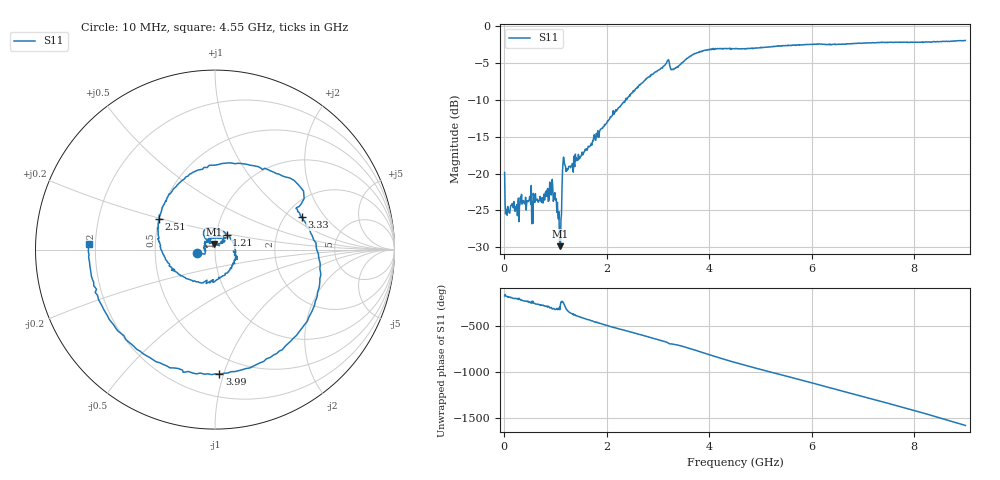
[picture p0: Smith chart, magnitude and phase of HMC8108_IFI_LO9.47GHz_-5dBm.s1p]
! Analog Devices, Inc.
! 1 Analog Way
! Wilmington, MA 01887
! http://www.analog.com
! Date:  2021-09-07 NN
! Board Name:  EV1HMC8108LC5 Revision A with HMC8108LC5 installed
! File Description:  S-Parameters for evaluation board without connectors or board loss de-embedded
! File Generation:  Calibrated Network Analyzer
! Chip Part Number:  HMC8108
! Chip Description:  X-Band, GaAs, MMIC, Low Noise Converter
! Chip Frequency:  9 to 10 GHz
! Chip Package:  LCC, 5 x 5 x 1.12 mm
! Chip State:
!  Temperature:  25C
!  LO Frequency:  9.47GHz
!  LO Power:  -5dBm
! Note:
!  Analog Devices supplies this data as a sample of measured data at the evaluation board
!  ports for this product.  Your particular data for this product may vary.
!  Analog Devices reserves the right to change this data at anytime.
!  All lines below in this file are as is from the Network Analyzer.
!Keysight Technologies,N5245A,MY49151104,A.10.65.16
!Date: Thursday, August 19, 2021 13:48:33
!Correction: S22(Full 2 Port(1,2))
!S1P File: Measurement: S22:
# Hz S  dB  R 50
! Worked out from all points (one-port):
!   900 points, 10 MHz to 9 GHz, reference 50 ohm
!   lowest |S11| = -29.8 dB at 1.1 GHz (marker M1), VSWR 1.07, Z = 49.4 + j3.15 ohm
!   |S11| at or under -10 dB: start of sweep to 2.373 GHz
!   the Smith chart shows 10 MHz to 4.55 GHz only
!   S11 on the Smith chart (normalised r, x): 10 MHz: 0.82, -0.03; 1.21 GHz: 1.12, +0.18; 2.51 GHz: 0.50, +0.19; 3.33 GHz: 2.44, +1.21; 3.99 GHz: 0.36, -0.97; 4.55 GHz: 0.18, +0.02
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1e7  -19.85 -170.0
7e7  -24.45 176.1
9.3e8  -21.88 54.5
1.1e9  -29.84 98.7
1.14e9  -19.62 127.7
1.21e9  -19.71 51.5
1.79e9  -15.47 -93.2
2.26e9  -10.88 -172.6
2.51e9  -9.01 151.6
2.96e9  -6.18 79.7
3.33e9  -5.75 20.6
3.39e9  -5.59 13.8
3.68e9  -3.87 -32.5
3.99e9  -3.17 -87.9
4.51e9  -3.03 -176.6
4.55e9  -3.08 177.4
5.11e9  -2.86 93.4
5.63e9  -2.56 18.0
5.92e9  -2.48 -24.7
6.24e9  -2.46 -72.9
6.5e9  -2.48 -111.7
6.76e9  -2.38 -151.0
7.07e9  -2.29 162.9
7.41e9  -2.19 112.3
7.88e9  -2.21 41.2
8.22e9  -2.16 -12.6
8.55e9  -2.06 -66.9
9e9  -1.94 -140.8
